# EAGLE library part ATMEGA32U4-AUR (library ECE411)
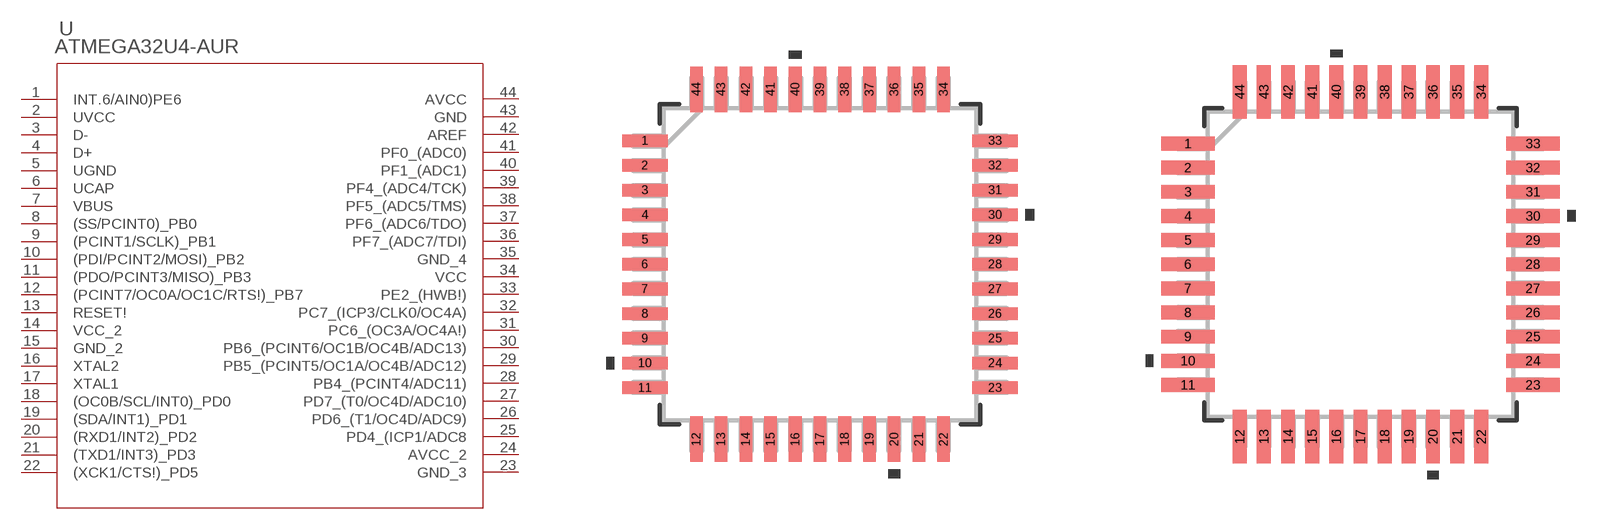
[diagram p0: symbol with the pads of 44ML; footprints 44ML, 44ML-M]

Designator prefix U

## ATMEGA32U4-AUR (MANUFACTURER_PART_NUMBER: ATMEGA32U4AUR; VENDOR: Atmel)  [44ML]
1  INT.6/AIN0)PE6
2  UVCC  pwr
3  D-  pas
4  D+  pas
5  UGND  pwr
6  UCAP  pwr
7  VBUS  pwr
8  (SS/PCINT0)_PB0
9  (PCINT1/SCLK)_PB1
10  (PDI/PCINT2/MOSI)_PB2
11  (PDO/PCINT3/MISO)_PB3
12  (PCINT7/OC0A/OC1C/RTS!)_PB7
13  RESET!  in
14  VCC_2  pwr
15  GND_2  pwr
16  XTAL2  out
17  XTAL1  in
18  (OC0B/SCL/INT0)_PD0
19  (SDA/INT1)_PD1
20  (RXD1/INT2)_PD2
21  (TXD1/INT3)_PD3
22  (XCK1/CTS!)_PD5
23  GND_3  pwr
24  AVCC_2  pwr
25  PD4_(ICP1/ADC8
26  PD6_(T1/OC4D/ADC9)
27  PD7_(T0/OC4D/ADC10)
28  PB4_(PCINT4/ADC11)
29  PB5_(PCINT5/OC1A/OC4B/ADC12)
30  PB6_(PCINT6/OC1B/OC4B/ADC13)
31  PC6_(OC3A/OC4A!)
32  PC7_(ICP3/CLK0/OC4A)
33  PE2_(HWB!)
34  VCC  pwr
35  GND_4  pwr
36  PF7_(ADC7/TDI)
37  PF6_(ADC6/TDO)
38  PF5_(ADC5/TMS)
39  PF4_(ADC4/TCK)
40  PF1_(ADC1)
41  PF0_(ADC0)
42  AREF  pas
43  GND  pwr
44  AVCC  pwr

## ATMEGA32U4-AUR44ML-M (MANUFACTURER_PART_NUMBER: ATMEGA32U4AUR; VENDOR: Atmel)  [44ML-M]
Pads as for 44ML

## ATMEGA32U4-AUR44ML-L (MANUFACTURER_PART_NUMBER: ATMEGA32U4AUR; VENDOR: Atmel)  [44ML-L]
Pads as for 44ML

## Footprint 44ML (pad centres in mm)
smd 1.473 x 0.406: 1 -5.664,4; 2 -5.664,3.2; 3 -5.664,2.4; 4 -5.664,1.6; 5 -5.664,0.8; 6 -5.664,0; 7 -5.664,-0.8; 8 -5.664,-1.6; 9 -5.664,-2.4; 10 -5.664,-3.2; 11 -5.664,-4; 23 5.664,-4; 24 5.664,-3.2; 25 5.664,-2.4; 26 5.664,-1.6; 27 5.664,-0.8; 28 5.664,0; 29 5.664,0.8; 30 5.664,1.6; 31 5.664,2.4; 32 5.664,3.2; 33 5.664,4
smd 0.406 x 1.473: 12 -4,-5.664; 13 -3.2,-5.664; 14 -2.4,-5.664; 15 -1.6,-5.664; 16 -0.8,-5.664; 17 0,-5.664; 18 0.8,-5.664; 19 1.6,-5.664; 20 2.4,-5.664; 21 3.2,-5.664; 22 4,-5.664; 34 4,5.664; 35 3.2,5.664; 36 2.4,5.664; 37 1.6,5.664; 38 0.8,5.664; 39 0,5.664; 40 -0.8,5.664; 41 -1.6,5.664; 42 -2.4,5.664; 43 -3.2,5.664; 44 -4,5.664

## Footprint 44ML-M (pad centres in mm)
smd 1.778 x 0.457: 1 -5.715,4; 2 -5.715,3.2; 3 -5.715,2.4; 4 -5.715,1.6; 5 -5.715,0.8; 6 -5.715,0; 7 -5.715,-0.8; 8 -5.715,-1.6; 9 -5.715,-2.4; 10 -5.715,-3.2; 11 -5.715,-4; 23 5.715,-4; 24 5.715,-3.2; 25 5.715,-2.4; 26 5.715,-1.6; 27 5.715,-0.8; 28 5.715,0; 29 5.715,0.8; 30 5.715,1.6; 31 5.715,2.4; 32 5.715,3.2; 33 5.715,4
smd 0.457 x 1.778: 12 -4,-5.715; 13 -3.2,-5.715; 14 -2.4,-5.715; 15 -1.6,-5.715; 16 -0.8,-5.715; 17 0,-5.715; 18 0.8,-5.715; 19 1.6,-5.715; 20 2.4,-5.715; 21 3.2,-5.715; 22 4,-5.715; 34 4,5.715; 35 3.2,5.715; 36 2.4,5.715; 37 1.6,5.715; 38 0.8,5.715; 39 0,5.715; 40 -0.8,5.715; 41 -1.6,5.715; 42 -2.4,5.715; 43 -3.2,5.715; 44 -4,5.715

## Footprint 44ML-L (pad centres in mm)
smd 1.168 x 0.356: 1 -5.613,4; 2 -5.613,3.2; 3 -5.613,2.4; 4 -5.613,1.6; 5 -5.613,0.8; 6 -5.613,0; 7 -5.613,-0.8; 8 -5.613,-1.6; 9 -5.613,-2.4; 10 -5.613,-3.2; 11 -5.613,-4; 23 5.613,-4; 24 5.613,-3.2; 25 5.613,-2.4; 26 5.613,-1.6; 27 5.613,-0.8; 28 5.613,0; 29 5.613,0.8; 30 5.613,1.6; 31 5.613,2.4; 32 5.613,3.2; 33 5.613,4
smd 0.356 x 1.168: 12 -4,-5.613; 13 -3.2,-5.613; 14 -2.4,-5.613; 15 -1.6,-5.613; 16 -0.8,-5.613; 17 0,-5.613; 18 0.8,-5.613; 19 1.6,-5.613; 20 2.4,-5.613; 21 3.2,-5.613; 22 4,-5.613; 34 4,5.613; 35 3.2,5.613; 36 2.4,5.613; 37 1.6,5.613; 38 0.8,5.613; 39 0,5.613; 40 -0.8,5.613; 41 -1.6,5.613; 42 -2.4,5.613; 43 -3.2,5.613; 44 -4,5.613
